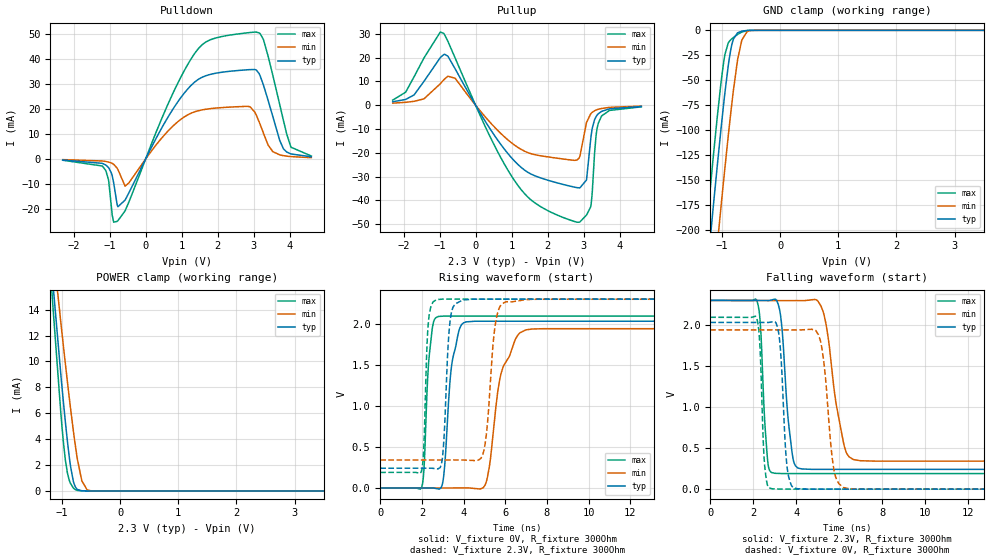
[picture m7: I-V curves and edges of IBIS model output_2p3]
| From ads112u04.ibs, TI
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|   output_2p3 Model
[Model]   output_2p3
Model_type   3-state
Polarity   Non-Inverting
Vmeas = 1.15
Vref = 0
Cref = 2pF
Rref = 100000
|   typ   min   max
C_comp   1.504E-12   1.49024E-12   1.51372E-12
|C_comp_pullup   1.3831E-12   1.3831E-12   1.38433E-12
|C_comp_pulldown   1.25791E-12   1.21354E-12   1.34289E-12
| Where Nom  PVT is Nominal Process, 2.3V, 27C
|   Fast PVT is Strong Process,  2.301V, -40C
|   Slow PVT is Weak Process,   2.299, 125C
[Voltage Range]   2.3   2.299   2.301
[Temperature Range]   27   125   -40
[Pullup Reference]   2.3   2.299   2.301
[Pulldown Reference]   -0   0   -0
[Power Clamp Reference]   2.3   2.299   2.301
[GND Clamp Reference]   0   0   0
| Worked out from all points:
|   slope of the pulldown table from 0 to 0.345 V, typ, clamps not added: 35.7 ohm
|   slope of the pullup table from 0 to 0.345 V, typ, clamps not added: 40.1 ohm
|   GND clamp passes 1 mA (typ) near -0.67 V on its own axis
|   POWER clamp passes 1 mA (typ) near -0.81 V on its own axis
|   falling waveform, V_fixture 2.3V, R_fixture 300Ohm: 20-80 % time 350ps typ, 628ps min, 230ps max; typ from 2.3 V to 0.241 V
|   rising waveform, V_fixture 0V, R_fixture 300Ohm: 20-80 % time 389ps typ, 772ps min, 244ps max; typ from 0 V to 2.03 V
|   rising waveform, V_fixture 2.3V, R_fixture 300Ohm: 20-80 % time 229ps typ, 353ps min, 164ps max; typ from 0.241 V to 2.3 V
|   falling waveform, V_fixture 0V, R_fixture 300Ohm: 20-80 % time 239ps typ, 389ps min, 173ps max; typ from 2.03 V to 0 V
[Pulldown]
|   Voltage   I(typ)   I(min)   I(max)
-2.3V     -376.1uA   -210.5uA   -460.9uA
-1.196V   -1.735mA   -769.2uA   -2.832mA
-1.03V    -3.335mA   -1.185mA   -8.202mA
-947.6mV  -5.602mA   -1.585mA   -19.24mA
-788.9mV  -18.22mA   -3.604mA   -24.82mA
-568.1mV  -16.33mA   -10.79mA   -20.63mA
1.371V    30.78mA    18.88mA    42.25mA
3.041V    35.64mA    18.46mA    50.6mA
3.275V    29.31mA    10.2mA     47.43mA
3.724V    7.421mA    1.678mA    21.68mA
4.034V    2.043mA    988.6uA    4.737mA
4.6V      908.2uA    565.3uA    1.225mA
[GND Clamp]
|   Voltage   I(typ)   I(min)   I(max)
-2.3V     -915.1mA   -992.7mA   -866.9mA
-1.389V   -326mA     -406.1mA   -275.6mA
-1.161V   -184.4mA   -264.3mA   -134.3mA
-1.079V   -134.9mA   -214.1mA   -86.05mA
-1.017V   -99.15mA   -177.1mA   -52.92mA
-947.6mV  -62.01mA   -137.2mA   -24.04mA
-892.4mV  -35.96mA   -106.4mA   -12.86mA
-830.3mV  -14.47mA   -73.75mA   -8.485mA
-726.8mV  -2.419mA   -28.25mA   -3.961mA
-657.8mV  -817.6uA   -9.695mA   -1.753mA
-492.2mV  -20.36uA   -193.5uA   -36.73uA
4.6V      0A         0A         0A
[Pullup]
|   Voltage   I(typ)   I(min)   I(max)
-2.3V     1.451mA    876.4uA    2.144mA
-1.707V   4.343mA    1.629mA    11.97mA
-885.5mV  21.27mA    10.62mA    30.22mA
-568.1mV  15.34mA    11.32mA    19.89mA
425.5mV   -10.49mA   -7.592mA   -13.97mA
1.171V    -24.86mA   -17.71mA   -33.66mA
2.82V     -34.68mA   -23.04mA   -49.21mA
3.075V    -31.54mA   -7.52mA    -46.26mA
3.192V    -14.78mA   -3.694mA   -42.88mA
3.344V    -4.806mA   -2.045mA   -12.81mA
3.496V    -2.603mA   -1.37mA    -4.538mA
4.6V      -539.4uA   -365.9uA   -683.8uA
[POWER Clamp]
|   Voltage   I(typ)   I(min)   I(max)
-2.3V     81.53mA    72.04mA    93.59mA
-1.217V   19.41mA    21.51mA    18.31mA
-1.161V   16.41mA    19.09mA    14.7mA
-1.148V   15.67mA    18.49mA    13.82mA
-1.017V   8.893mA    12.92mA    5.903mA
-940.7mV  5.33mA     9.824mA    2.391mA
-906.2mV  3.864mA    8.457mA    1.398mA
-851mV    1.876mA    6.348mA    565.2uA
-768.2mV  300.5uA    3.472mA    95.99uA
-657.8mV  12.87uA    779.7uA    3.786uA
-519.8mV  252.1nA    24.76uA    21.56nA
4.6V      0A         0A         0A
[Ramp]
R_load = 300
|   typ   min   max
dV/dt_r   1.21887/3.89411e-10   1.16426/7.705e-10   1.25651/2.44438e-10
dV/dt_f   1.23544/3.51003e-10   1.17475/6.29321e-10   1.26664/2.29549e-10
[Falling Waveform]
V_fixture = 2.3V
V_fixture_min = 2.299V
V_fixture_max = 2.301V
R_fixture = 300Ohm
C_fixture = 0F
|   Time   V(typ)   V(min)   V(max)
0s        2.3V       2.299V     2.301V
2.167ns   2.299V     2.298V     2.297V
2.67ns    2.299V     2.298V     348.6mV
3.003ns   2.315V     2.298V     193.4mV
3.31ns    2.03V      2.298V     190.4mV
3.817ns   426.9mV    2.298V     190.2mV
4.274ns   246mV      2.298V     190.2mV
5.254ns   241.3mV    2.161V     190.2mV
6.713ns   241.3mV    357.6mV    190.2mV
50ns      240.9mV    341.1mV    189.9mV
[Rising Waveform]
V_fixture = 0V
V_fixture_min = 0V
V_fixture_max = 0V
R_fixture = 300Ohm
C_fixture = 0F
|   Time   V(typ)   V(min)   V(max)
0s        -18.38nV   -32.18nV   -43.64nV
1.981ns   621.6uV    297.1uV    3.624mV
2.356ns   739.2uV    353.3uV    1.625V
2.787ns   -11.28mV   417.9uV    2.089V
3.454ns   1.54V      517.9uV    2.094V
4.11ns    2.023V     616.3uV    2.094V
5.037ns   2.031V     38.59mV    2.094V
5.806ns   2.031V     1.4V       2.094V
6.996ns   2.031V     1.926V     2.094V
50ns      2.031V     1.94V      2.094V
[Rising Waveform]
V_fixture = 2.3V
V_fixture_min = 2.299V
V_fixture_max = 2.301V
R_fixture = 300Ohm
C_fixture = 0F
|   Time   V(typ)   V(min)   V(max)
0s        240.9mV    341.1mV    189.9mV
1.969ns   241.2mV    341.2mV    195.4mV
2.311ns   241.3mV    341.2mV    2.021V
2.699ns   234.7mV    341.2mV    2.294V
3ns       406.3mV    341.2mV    2.301V
3.401ns   2.118V     341.2mV    2.301V
3.965ns   2.29V      341.2mV    2.301V
4.979ns   2.3V       458.8mV    2.301V
6.067ns   2.3V       2.269V     2.301V
50ns      2.3V       2.299V     2.301V
[Falling Waveform]
|Gnd
V_fixture = 0V
V_fixture_min = 0V
V_fixture_max = 0V
R_fixture = 300Ohm
C_fixture = 0F
|   Time   V(typ)   V(min)   V(max)
0s        2.031V     1.94V      2.094V
2.152ns   2.031V     1.94V      2.092V
2.533ns   2.031V     1.94V      279.1mV
2.887ns   2.039V     1.94V      4.17mV
3.587ns   243.5mV    1.94V      249.7uV
4.068ns   4.658mV    1.94V      249.6uV
5.116ns   375.5uV    1.816V     249.3uV
5.746ns   375.3uV    248.8mV    249.1uV
6.459ns   375uV      6.25mV     249uV
50ns      -52.05nV   -5.827nV   -44nV
